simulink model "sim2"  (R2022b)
settings: Solver=VariableStepAuto  StartTime=0.0  StopTime=10.0  MaxStep=0.05  RelTol=1e-3

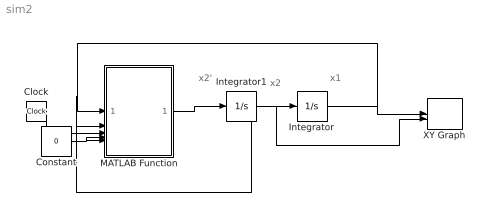
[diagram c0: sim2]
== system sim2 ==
  note: x2'
  note: x2
  note: x1
  Clock : Clock
  Constant : Constant  Value=0
  Integrator : Integrator
  Integrator1 : Integrator
  MATLAB Function : MATLAB Function  TreatAsAtomicUnit=on
  XY Graph : Record  FileSettingsInternal="{\"entries\":[{\"content\":{\"excelSettings\":{\"content\":{},\"type\":\"Streamout.ExcelSettings\"}},\"type\":\"Streamout.FileSettingStorage\",\"uuid\":\"1e22f633-acec-4a21-a45e-44c5d5d399ff\"}],\"packageUris\":[\"http://schema.mathworks.com/mf0/streamout_blocks/R2020a\"],\"version\":\"1.0\"}"  Layout=[1 1]  SignalsInternal="{\"entries\":[{\"content\":{\"signals\":[{\"content\":{\"blockPath\":[\"untitled/XY Graph\"],\"channel\":[],\"dimensions\":[1],\"domain\":\"untitled/XY Graph\",\"lineColor\":\"#a2142f\",\"plots\":[1],\"port\":1,\"sid\":[\"\"],\"signalID\":253,\"signalName\":\"Integrator\"},\"type\":\"RecordBlkView.Signal\",\"uuid\":\"782dd91b-d7c6-48cb-9093-6d0edb0b0fdb\"},{\"content\":{\"blockPath\":[\"untitled/XY Graph\"],\"channel\":[],\"dimensions\":[1],\"domain\":\"u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"  VisualizationBindings="{\"xyplotplugin\":{\"info\":[{\"series\":[{\"bindingParametersList\":[{\"parameter\":\"X-Axis\",\"signalID\":253,\"signalName\":\"Integrator\"},{\"parameter\":\"Y-Axis\",\"signalID\":257,\"signalName\":\"Integrator1\"}],\"seriesID\":13253}],\"subplotID\":1}]}}"  CompatibilityTag=XY
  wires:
  Integrator1/1 -> XY Graph/2, Integrator/1, MATLAB Function/2(x2)
  Integrator/1 -> MATLAB Function/1(x1), XY Graph/1
  MATLAB Function/1(x2dot) -> Integrator1/1
  Clock/1 -> MATLAB Function/3(t)
  Constant/1 -> MATLAB Function/5(d), MATLAB Function/4(u)

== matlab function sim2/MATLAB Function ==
function x2dot  = fcn(x1,x2,t,u,d)

x2dot = -0.1*x2-x1^3+12*cos(t)+u+d;
